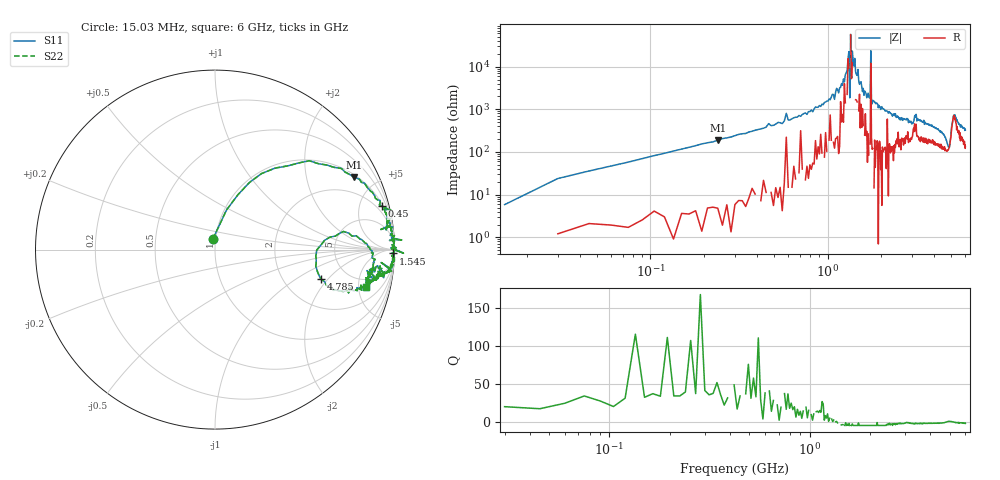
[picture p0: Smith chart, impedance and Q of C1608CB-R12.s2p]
!	Network	Analyzer	HP8753E.07.74:	Oct	30	2002	Serial	No.	JP38451487
!	Hewlett-Packard
!	7	Sep	2009	9:55:44
!	Frequency	S11	S21	S12	S22
#	HZ	S	RI	R	50
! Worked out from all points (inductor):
!   400 points, 15.03 MHz to 6 GHz, reference 50 ohm
!   read as one part in series: L = 124 nH near 45.03 MHz
!   highest Q = 39.1 at 240 MHz (marker M1), where L = 125 nH
!   self-resonance near 1.32 GHz
!   S11 on the Smith chart (normalised r, x): 15.03 MHz: 0.97, +0.11; 450 MHz: 1.22, +7.65; 1.545 GHz: 27, -85; 4.785 GHz: 3.21, -1.66; 6 GHz: 3.68, -6.02
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1.502992e7  -0.0121 0.0582  1.01 -0.0582  1.01 -0.0582  -0.0121 0.0582
6.00297e7  0.191 0.373  0.809 -0.373  0.809 -0.373  0.191 0.373
2.400288e8  0.775 0.405  0.225 -0.405  0.225 -0.405  0.775 0.405
4.500278e8  0.93 0.241  0.0701 -0.241  0.0701 -0.241  0.93 0.241
1.020025e9  0.991 0.0558  0.00928 -0.0558  0.00928 -0.0558  0.991 0.0558
1.245024e9  0.98 0.00922  0.0202 -0.00922  0.0202 -0.00922  0.98 0.00922
1.320023e9  0.998 0.00403  0.00186 -0.00403  0.00186 -0.00403  0.998 0.00403
1.335023e9  1.05 -0.0198  -0.0529 0.0198  -0.0529 0.0198  1.05 -0.0198
1.350023e9  0.998 -0.000244  0.00174 0.000244  0.00174 0.000244  0.998 -0.000244
1.365023e9  0.983 0.00479  0.0174 -0.00479  0.0174 -0.00479  0.983 0.00479
1.380023e9  0.998 -0.00363  0.00232 0.00363  0.00232 0.00363  0.998 -0.00363
1.545022e9  0.993 -0.0212  0.00708 0.0212  0.00708 0.0212  0.993 -0.0212
1.740021e9  0.993 -0.0535  0.00739 0.0535  0.00739 0.0535  0.993 -0.0535
1.755021e9  0.998 -0.00363  0.00217 0.00363  0.00217 0.00363  0.998 -0.00363
1.770021e9  0.99 -0.0556  0.0101 0.0556  0.0101 0.0556  0.99 -0.0556
1.785021e9  0.988 -0.073  0.0118 0.073  0.0118 0.073  0.988 -0.073
2.01002e9  0.984 -0.0877  0.0164 0.0877  0.0164 0.0877  0.984 -0.0877
3.015015e9  0.886 -0.147  0.114 0.147  0.114 0.147  0.886 -0.147
4.00501e9  0.863 -0.191  0.137 0.191  0.137 0.191  0.863 -0.191
4.785006e9  0.589 -0.162  0.411 0.162  0.411 0.162  0.589 -0.162
5.010005e9  0.787 0.0768  0.213 -0.0768  0.213 -0.0768  0.787 0.0768
6e9  0.839 -0.207  0.161 0.207  0.161 0.207  0.839 -0.207
